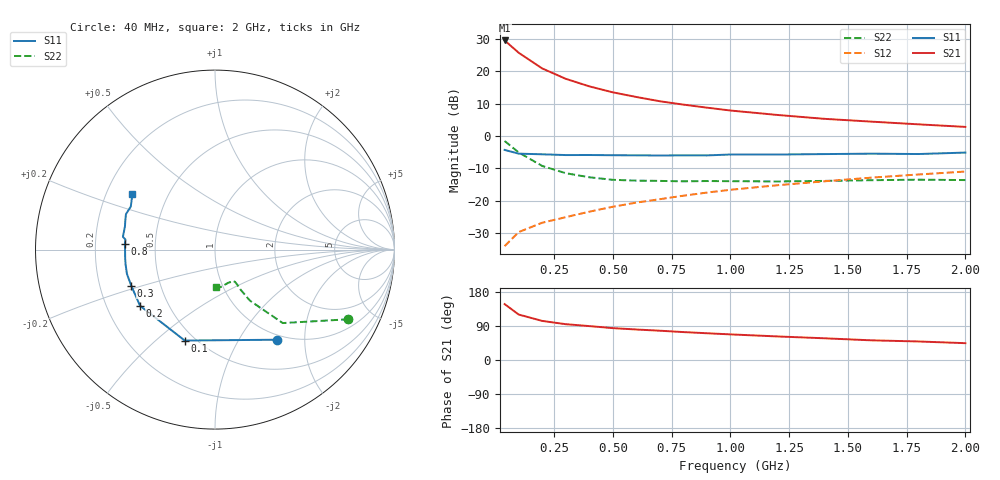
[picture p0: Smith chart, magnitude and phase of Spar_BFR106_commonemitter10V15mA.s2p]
! Filename:  BFR106E.S2P  Version:  2.0
! NXP part #: BFR106  Date: Jun 1990
! Bias condition: Vce=10V, Ic=15mA
#  MHz  S  MA  R  50
! Freq  S11  S21  S12  S22  !GUM [dB]
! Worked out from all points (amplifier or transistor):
!   16 points, 40 MHz to 2 GHz, reference 50 ohm
!   highest |S21| = 29.5 dB at 40 MHz (marker M1)
!   |S21| within 3 dB of that: start of sweep to 87.44 MHz
!   unconditionally stable (mu >= 1): 459.4 MHz to 1.846 GHz
!   at 200 MHz: K = 0.71, MSG = 23.8 dB, |S12| = -26.7 dB
!   at 800 MHz: K = 1.07, MAG = 12.4 dB, |S12| = -18.4 dB
!   at 2 GHz: K = 0.97, MSG = 6.9 dB, |S12| = -11.0 dB
!   S11 on the Smith chart (normalised r, x): 40 MHz: 0.92, -1.48; 100 MHz: 0.44, -0.62; 200 MHz: 0.35, -0.30; 300 MHz: 0.34, -0.18; 800 MHz: 0.33, +0.03; 2 GHz: 0.31, +0.28
40  0.61 -55.4  29.73 147.5  0.02 67.8  0.838 -27.6
100  0.534 -108.4  19.21 119.9  0.033 54.9  0.557 -47.3
200  0.522 -143.2  11.01 103.1  0.046 54.8  0.345 -55.6
300  0.508 -156.7  7.618 94.5  0.056 56.7  0.267 -57.4
400  0.509 -164.6  5.828 89.5  0.068 61.2  0.231 -57.6
500  0.505 -170.5  4.713 84.1  0.081 63.7  0.211 -58.2
600  0.503 -174.3  3.996 80.5  0.094 65.8  0.205 -59.5
700  0.501 -178.9  3.435 77.3  0.106 66.7  0.203 -60.6
800  0.503 176.5  3.048 73.7  0.12 67.1  0.2 -61.6
900  0.502 173.6  2.737 70.6  0.134 68.5  0.202 -62.7
1000  0.518 172.1  2.472 67.6  0.148 68.3  0.201 -64.0
1200  0.518 165.6  2.111 62.2  0.174 68.4  0.199 -68.3
1400  0.526 161.7  1.84 57.3  0.2 67.7  0.203 -73.8
1600  0.534 158.3  1.665 51.9  0.228 67.8  0.208 -77.8
1800  0.527 152.9  1.513 48.9  0.255 66.7  0.212 -83.1
2000  0.555 146.0  1.381 44.4  0.283 65.8  0.209 -88.1
